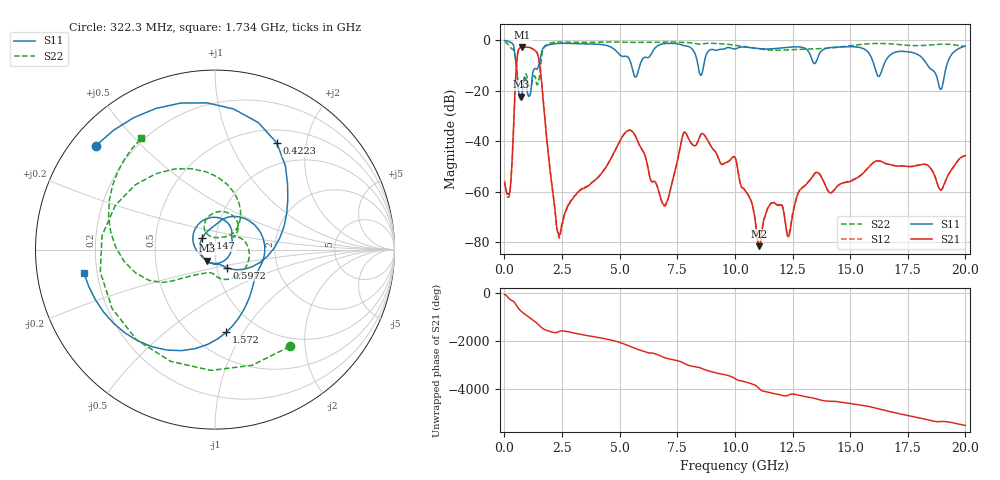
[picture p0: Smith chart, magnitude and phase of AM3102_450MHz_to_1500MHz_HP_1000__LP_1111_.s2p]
!Agilent Technologies,E8364B,MY43040894,A.07.50.67
!Agilent E8364B: A.07.50.67
!Date: Thursday, January 11, 2018 06:00:29
!Correction: S11(Full 2 Port(1,2))
!S21(Full 2 Port(1,2))
!S12(Full 2 Port(1,2))
!S22(Full 2 Port(1,2))
!S2P File: Measurements: S11, S21, S12, S22:
# Hz S  dB  R 50
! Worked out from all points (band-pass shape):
!   1601 points, 10 MHz to 20 GHz, reference 50 ohm
!   highest |S21| = -2.68 dB at 784.6 MHz (marker M1); lowest = -81.5 dB at 11.05 GHz (marker M2)
!   |S21| within 3 dB of the highest: 570.4 MHz to 1.449 GHz (878.5 MHz wide, 87 % of centre)
!   lowest |S11| = -22.3 dB at 709.6 MHz (marker M3), VSWR 1.17, Z = 45.3 - j5.61 ohm
!   |S11| at or under -10 dB: 515 MHz to 1.487 GHz (972.3 MHz wide, 97.1 % of centre); 16.05 GHz to 16.45 GHz (400.8 MHz wide, 2.47 % of centre); 18.37 GHz to 19.19 GHz (819.2 MHz wide, 4.36 % of centre)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
!   |S22| runs from -23.5 to -0.6 dB; largest |S21 - S12| = 0.0015
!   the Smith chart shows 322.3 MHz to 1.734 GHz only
!   S11 on the Smith chart (normalised r, x): 322.3 MHz: 0.07, +0.37; 422.3 MHz: 0.68, +1.52; 597.2 MHz: 1.11, -0.23; 1.147 GHz: 0.86, +0.11; 1.572 GHz: 0.72, -0.85; 1.734 GHz: 0.15, -0.09
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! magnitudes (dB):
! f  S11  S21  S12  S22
! 10 MHz  -0.1  -56.8  -55.6  -0.6
! 322.3 MHz  -1.1  -50.0  -50.0  -3.3
! 422.3 MHz  -3.3  -28.3  -28.3  -4.3
! 597.2 MHz  -18.5  -4.2  -4.2  -17.4
! 709.6 MHz  -22.3  -2.8  -2.8  -23.5
! 784.6 MHz  -19.8  -2.7  -2.7  -20.9
! 1.147 GHz  -20.3  -3.0  -3.0  -18.1
! 1.572 GHz  -6.7  -12.6  -12.6  -10.6
! 1.734 GHz  -2.6  -28.9  -28.9  -2.6
! 2.334 GHz  -1.2  -76.5  -76.6  -0.7
! 3.346 GHz  -1.4  -59.0  -58.7  -0.8
! 5.432 GHz  -7.7  -35.6  -35.6  -0.8
! 6.682 GHz  -2.0  -59.3  -59.3  -0.7
! 7.031 GHz  -1.2  -64.4  -64.7  -0.7
! 7.819 GHz  -2.2  -36.3  -36.3  -0.9
! 10.01 GHz  -3.4  -46.4  -46.4  -2.0
! 11.05 GHz  -3.3  -81.5  -81.2  -3.4
! 12.34 GHz  -2.7  -77.5  -76.8  -3.8
! 13.34 GHz  -7.5  -54.4  -54.4  -3.4
! 16.68 GHz  -6.3  -49.1  -49.1  -1.3
! 18.93 GHz  -19.4  -59.2  -59.4  -1.5
! 20 GHz  -2.3  -45.7  -45.6  -2.4
